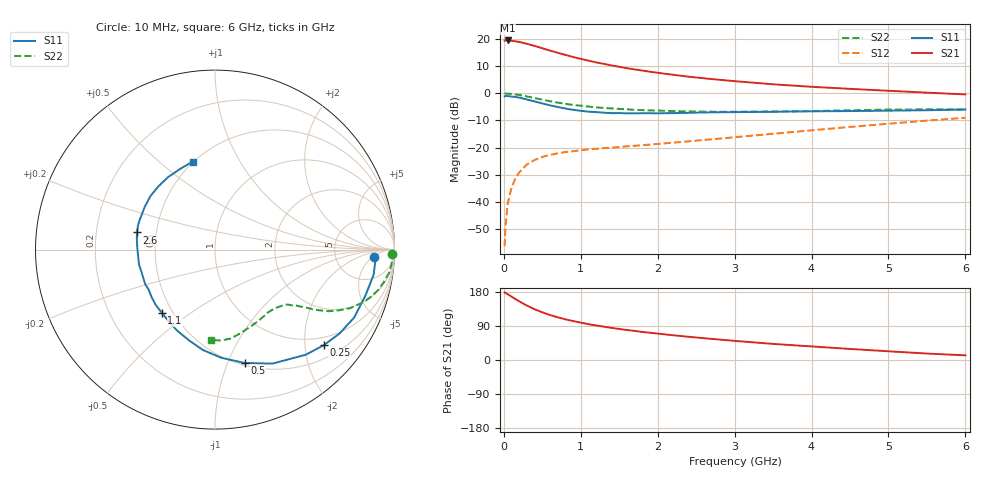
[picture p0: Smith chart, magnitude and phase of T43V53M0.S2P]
! Infineon Technologies  Discrete & RF Semiconductors
! BFR182T
! Si NPN RF Bipolar Junction Transistor in SC75
! VCE = 3.5 V  IC = 3 mA
! Common Emitter S-Parameters:  October  1999
# GHz  S  MA  R  50
!  f  S11  S21  S12  S22
! GHz  MAG  ANG  MAG  ANG  MAG  ANG  MAG  ANG
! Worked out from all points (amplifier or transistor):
!   36 points, 10 MHz to 6 GHz, reference 50 ohm
!   highest |S21| = 19.6 dB at 50 MHz (marker M1)
!   |S21| within 3 dB of that: start of sweep to 514.1 MHz
!   unconditionally stable (mu >= 1): 1.728 GHz to 4.197 GHz
!   at 250 MHz: K = 0.20, MSG = 23.2 dB, |S12| = -27.7 dB
!   at 1.4 GHz: K = 0.89, MSG = 15.2 dB, |S12| = -20.1 dB
!   at 6 GHz: K = 0.83, MSG = 4.3 dB, |S12| = -9.0 dB
!   lowest NFmin = 1.10 dB at 450 MHz
!   S11 on the Smith chart (normalised r, x): 10 MHz: 14, -6; 250 MHz: 0.79, -2.42; 500 MHz: 0.52, -1.15; 1.1 GHz: 0.44, -0.39; 2.6 GHz: 0.39, +0.09; 6 GHz: 0.49, +0.65
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0.01  0.886 -2.8  9.528 178.0  0.0015 88.2  0.9864 -1.5
0.02  0.897 -2.3  9.52 177.6  0.0033 97.9  0.9999 -1.5
0.05  0.895 -8.9  9.552 173.4  0.0091 86.4  0.9898 -3.8
0.15  0.8629 -26.0  9.224 160.8  0.027 75.1  0.9594 -10.7
0.2  0.8368 -34.0  8.965 154.8  0.0347 72.7  0.9371 -13.9
0.25  0.8062 -41.4  8.628 149.1  0.0412 68.1  0.9092 -16.7
0.3  0.7739 -49.2  8.273 143.7  0.0485 65.6  0.8812 -19.2
0.4  0.7115 -63.2  7.575 133.8  0.0589 59.2  0.8211 -23.4
0.5  0.6531 -75.3  6.858 125.8  0.067 55.2  0.7668 -26.2
0.6  0.6033 -86.8  6.208 118.7  0.073 51.8  0.7193 -28.5
0.7  0.563 -97.0  5.653 112.7  0.0782 49.7  0.6775 -30.0
0.8  0.5256 -106.1  5.168 107.3  0.0825 48.0  0.643 -31.3
0.9  0.4982 -115.1  4.723 102.8  0.0855 47.2  0.6138 -32.1
1.1  0.4601 -130.1  4.043 94.5  0.0925 46.2  0.5719 -33.7
1.5  0.4338 -153.9  3.111 81.9  0.1023 47.4  0.5189 -36.5
1.8  0.4309 -168.2  2.654 74.1  0.1105 49.1  0.4914 -39.2
2.2  0.4331 178.6  2.215 65.3  0.123 52.1  0.4734 -42.8
2.6  0.445 167.6  1.908 57.5  0.1382 54.7  0.4609 -47.5
3.5  0.458 148.8  1.478 42.5  0.1796 58.6  0.4653 -58.9
4.5  0.4725 132.2  1.217 29.2  0.2403 58.9  0.4874 -73.1
5.5  0.4897 113.5  1.035 17.0  0.3147 55.7  0.5073 -86.4
6  0.5055 104.3  0.96 12.3  0.3556 52.6  0.5038 -92.3
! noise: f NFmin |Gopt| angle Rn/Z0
0.45  1.1  0.37  30  0.33
0.9  1.2  0.35  61  0.26
1.8  1.85  0.27  133  0.2
